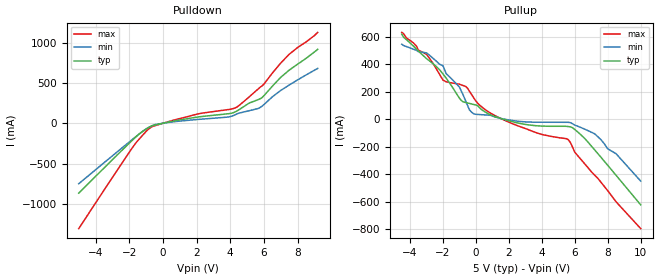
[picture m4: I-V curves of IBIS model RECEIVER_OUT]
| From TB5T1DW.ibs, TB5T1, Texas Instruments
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|   Receiver Output Model
[Model]   RECEIVER_OUT
Model_type   3-state
| Signals   AO,BO,CO,DO
Vmeas = 1.5V   |Reference voltage for timing measurements
Cref = 10pF   |Timing specification test load capacitance value
| variable   typ   min   max
C_comp   967fF   940fF   1007fF
|   typ   min   max
[Temperature Range]   25.0   -40.0   125.0
[Voltage range]   5.0V   4.5V   5.5V
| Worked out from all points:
|   slope of the pulldown table from 0 to 0.75 V, typ, clamps not added: 23 ohm
|   slope of the pullup table from 0 to 0.75 V, typ, clamps not added: 11.8 ohm
[Pulldown]
|   Voltage   I(typ)   I(min)   I(max)
-5V       -868mA     -752mA     -1.31A
-1.8V     -208mA     -199mA     -300mA
-800mV    -47.4mA    -46.5mA    -63.1mA
-300mV    -14.3mA    -9.76mA    -19.3mA
1.8V      69.3mA     42.6mA     102mA
3.9V      119mA      78.8mA     171mA
4.4V      153mA      116mA      202mA
5.7V      298mA      187mA      433mA
6V        342mA      232mA      486mA
7V        571mA      408mA      748mA
7.5V      660mA      475mA      857mA
9.2V      919mA      682mA      1.13A
[Pullup]
|   Voltage   I(typ)   I(min)   I(max)
| Note that the[Pullup]voltage table is referenced to Vcc
| and is calculated using Vtable=Vcc - Vmeasured.
-4.5V     620mA      547mA      633mA
-3V       442mA      484mA      474mA
-2V       331mA      390mA      286mA
-1.8V     299mA      332mA      273mA
-900mV    139mA      209mA      251mA
-400mV    116mA      70mA       206mA
-100mV    107mA      38.7mA     150mA
1.9V      -7.45mA    -2.48mA    -15.5mA
5.6V      -52.7mA    -21.7mA    -148mA
6V        -74.1mA    -42.5mA    -240mA
7.2V      -222mA     -105mA     -406mA
10V       -623mA     -450mA     -796mA
[Ramp]
|   typ   min   max
dV/dt_r   1.973V/1573ps   1.912V/2557ps   1.852V/1318ps
dV/dt_f   1.998V/1311ps   1.966V/1883ps   2.013V/994ps
R_load = 2000
